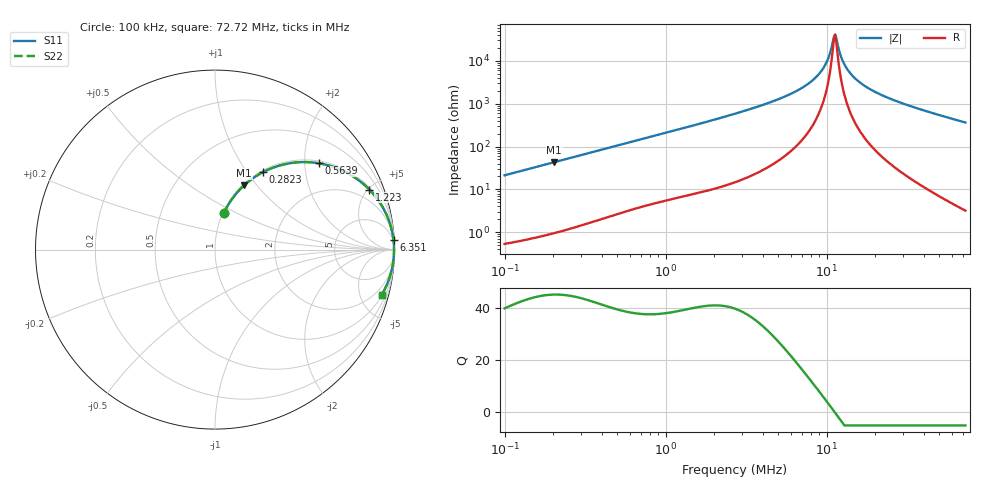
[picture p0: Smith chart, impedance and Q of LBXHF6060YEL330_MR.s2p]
! LBXHF6060YEL330_MR  S-PARAMETER MODEL  ( General Type )
! Model Generated by TAIYO YUDEN Corporation (http://www.ty-top.com)
! Version 1.0
! TAIYO YUDEN Control No. 201105NI43SB-FBB
! Copyright(c) 2020 TAIYO YUDEN CO.,LTD. All Rights Reserved.
! Product Description (link to TY-COMPAS)
! https://ds.yuden.co.jp/TYCOMPAS/or/detail?pn=LBXHF6060YEL330MMR&u=M
! Products Name : Inductors
! Characteristics :
!  Inductance : 33 uH , SRF(min) : 7.5 MHz , DC Resistance(max) : 0.216 Ohm
!  Rated Current : Saturation :1750 mA , Temp Rise : 750 mA
!  Case Size : 6.0 x 6.0 / 0.236 x 0.236 [mm/inch] , Thickness : 4.5 / 0.177 [mm/inch]
!  (Conditions: Temperature = 25 degC , DC Bias Current/Voltage = 0A / 0V)
! External Node Assignments :
!  1  o---GGG---o  2
! GND o---------o GND
! Frequency Range : 0.1MHz  -  72.722828MHz  [ 402 STEP ]
# MHz S RI R 50
! Freq[MHz].  S11 Real  S11 Imag  S21 Real  S21 Imag  S12 Real  S12 Imag  S22 Real  S22 Imag
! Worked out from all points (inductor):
!   401 points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, 100 kHz to 72.72 MHz, reference 50 ohm
!   read as one part in series: L = 33.8 uH near 103.3 kHz
!   highest Q = 45.3 at 203.1 kHz (marker M1), where L = 33.7 uH
!   self-resonance near 11.12 MHz
!   S11 on the Smith chart (normalised r, x): 100 kHz: 1.01, +0.43; 282.3 kHz: 1.03, +1.19; 563.9 kHz: 1.06, +2.36; 1.223 MHz: 1.13, +5.10; 6.351 MHz: 3, +38; 72.72 MHz: 1.06, -7.28
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0.1  0.0481 0.2018  0.9519 -0.2018  0.9519 -0.2018  0.0481 0.2018
0.203062  0.1617 0.3573  0.8383 -0.3573  0.8383 -0.3573  0.1617 0.3573
0.282301  0.2671 0.4313  0.7329 -0.4313  0.7329 -0.4313  0.2671 0.4313
0.30153  0.2928 0.4438  0.7072 -0.4438  0.7072 -0.4438  0.2928 0.4438
0.563882  0.5807 0.4807  0.4193 -0.4807  0.4193 -0.4807  0.5807 0.4807
0.909201  0.7763 0.4038  0.2237 -0.4038  0.2237 -0.4038  0.7763 0.4038
1.223024  0.8604 0.334  0.1396 -0.334  0.1396 -0.334  0.8604 0.334
2.741508  0.9687 0.1619  0.0313 -0.1619  0.0313 -0.1619  0.9687 0.1619
4.493812  0.9887 0.0904  0.0113 -0.0904  0.0113 -0.0904  0.9887 0.0904
6.351153  0.9946 0.0522  0.00538 -0.0522  0.00538 -0.0522  0.9946 0.0522
8.131398  0.9967 0.0287  0.00332 -0.0287  0.00332 -0.0287  0.9967 0.0287
8.976154  0.9972 0.0198  0.00284 -0.0198  0.00284 -0.0198  0.9972 0.0198
9.74678  0.9974 0.0125  0.00258 -0.0125  0.00258 -0.0125  0.9974 0.0125
10.24056  0.9975 0.00822  0.00247 -0.00822  0.00247 -0.00822  0.9975 0.00822
10.93806  0.9976 0.0025  0.00239 -0.0025  0.00239 -0.0025  0.9976 0.0025
11.30443  0.9976 -0.00036  0.00238 0.00036  0.00238 0.00036  0.9976 -0.00036
11.49219  0.9976 -0.00179  0.00238 0.00179  0.00238 0.00179  0.9976 -0.00179
12.6861  0.9975 -0.0104  0.00246 0.0104  0.00246 0.0104  0.9975 -0.0104
14.4731  0.9972 -0.022  0.00282 0.022  0.00282 0.022  0.9972 -0.022
17.9294  0.9959 -0.0418  0.00406 0.0418  0.00406 0.0418  0.9959 -0.0418
24.51857  0.9922 -0.0742  0.00784 0.0742  0.00784 0.0742  0.9922 -0.0742
72.72283  0.9279 -0.2544  0.0721 0.2544  0.0721 0.2544  0.9279 -0.2544
